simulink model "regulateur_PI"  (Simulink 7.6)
settings: Solver=ode45  StartTime=0.0  StopTime=10.0  RelTol=1e-3
InitFcn:
  | clc, close all
  | Kp=0.005;
  | R1=10e3;
  | R2=Kp*R1;
  | 
  | Ti=0.01;
  | C=Ti/R2;
libraries: fl_lib x6, nesl_utility x2, elec_lib x1

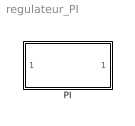
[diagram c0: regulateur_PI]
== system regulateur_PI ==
  PI : Subsystem

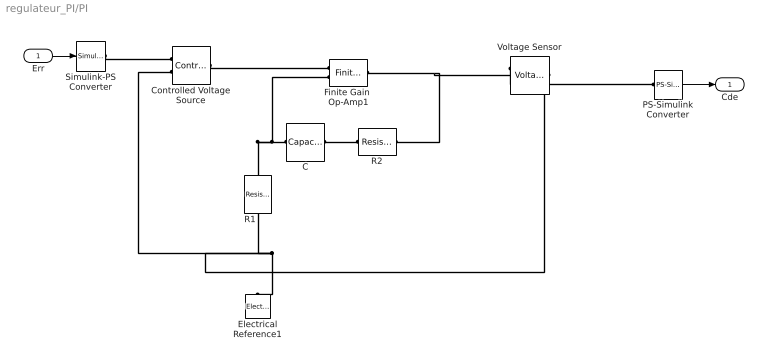
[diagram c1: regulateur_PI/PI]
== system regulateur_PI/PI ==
  Err : Inport
  C : fl_lib/Electrical/Electrical Elements/Capacitor  DialogController=NetworkEngine.DynNeDlgSource  SystemSampleTime=-1  c=C F  v0=0 V  r=1e-6 Ohm  g=0 1/Ohm  i_Log=off  v_Log=off  vc_Log=off  LocalVarNames=|i|v|vc  LocalVarDescs=|i|v|Internal variable for voltage across capacitor term  LocalVarLogging=[0 0 0]
  Controlled Voltage Source : fl_lib/Electrical/Electrical Sources/Controlled Voltage Source  DialogController=NetworkEngine.DynNeDlgSource  SystemSampleTime=-1  i_Log=off  v_Log=off  LocalVarNames=|i|v  LocalVarDescs=|i|v  LocalVarLogging=[0 0]
  Electrical Reference1 : fl_lib/Electrical/Electrical Elements/Electrical Reference  DialogController=NetworkEngine.DynNeDlgSource  SystemSampleTime=-1  i_Log=off  LocalVarNames=|i  LocalVarDescs=|i  LocalVarLogging=[]
  Finite Gain  Op-Amp1 : elec_lib/Integrated Circuits/Finite Gain Op-Amp  DialogController=NetworkEngine.DynNeDlgSource  SystemSampleTime=-1  A=1000  Rin=1e+6 Ohm  Rout=100 Ohm  Vmin=-15 V  Vmax=15 V  LocalVarLogging=[]
  PS-Simulink Converter : nesl_utility/PS-Simulink Converter  DialogController=NetworkEngine.DynNeUtilDlgSource  SystemSampleTime=-1  PhysicalDomain=network_engine_domain  LeftPortType=input  RightPortType=output  SubClassName=ps_output  Unit=1  AffineConversion=off
  R1 : fl_lib/Electrical/Electrical Elements/Resistor  DialogController=NetworkEngine.DynNeDlgSource  SystemSampleTime=-1  R=R1 Ohm  i_Log=off  v_Log=off  LocalVarNames=|current|voltage|power  LocalVarDescs=|Resistor current (A)|Voltage across resistor (V)|Power (W)  LocalVarLogging=[0 0 0]
  R2 : fl_lib/Electrical/Electrical Elements/Resistor  DialogController=NetworkEngine.DynNeDlgSource  SystemSampleTime=-1  R=R2 Ohm  i_Log=off  v_Log=off  LocalVarNames=|current|voltage|power  LocalVarDescs=|Resistor current (A)|Voltage across resistor (V)|Power (W)  LocalVarLogging=[0 0 0]
  Simulink-PS Converter : nesl_utility/Simulink-PS Converter  DialogController=NetworkEngine.DynNeUtilDlgSource  SystemSampleTime=-1  PhysicalDomain=network_engine_domain  LeftPortType=input  RightPortType=output  SubClassName=ps_input  Unit=1  AffineConversion=off  InputFilterTimeConstant=.001  UdotUserProvided=0
  Voltage Sensor : fl_lib/Electrical/Electrical Sensors/Voltage Sensor  DialogController=NetworkEngine.DynNeDlgSource  SystemSampleTime=-1  i1_Log=off  v1_Log=off  LocalVarNames=|i1|v1  LocalVarDescs=|i1|v1  LocalVarLogging=[0 0]
  Cde : Outport
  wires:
  Err/1 -> Simulink-PS Converter/1
  PS-Simulink Converter/1 -> Cde/1
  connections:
  C/LConn1 -- Finite Gain  Op-Amp1/LConn2 -- R1/RConn1
  C/RConn1 -- R2/LConn1
  Controlled Voltage Source/LConn1 -- Finite Gain  Op-Amp1/LConn1
  Simulink-PS Converter/RConn1 -- Controlled Voltage Source/RConn1
  Controlled Voltage Source/RConn2 -- R1/LConn1 -- Electrical Reference1/LConn1 -- Voltage Sensor/RConn2
  Finite Gain  Op-Amp1/RConn1 -- R2/RConn1 -- Voltage Sensor/LConn1
  Voltage Sensor/RConn1 -- PS-Simulink Converter/LConn1
